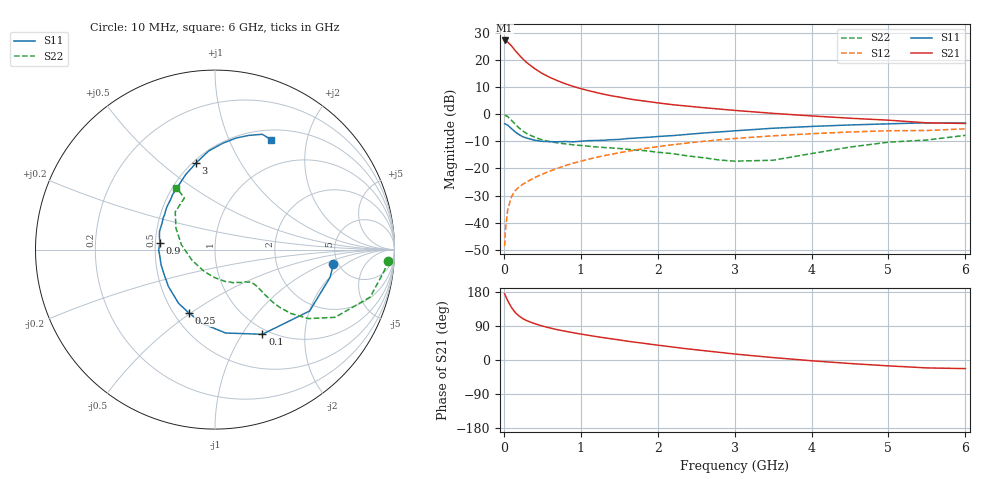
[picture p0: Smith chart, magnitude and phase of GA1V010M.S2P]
! Infineon Technologies  Discrete & RF Semiconductors
! BF775
! Si NPN RF Bipolar Junction Transistor in SOT23
! VCE = 1 V  IC = 10 mA
! Common Emitter S-Parameters:  May  1996
# GHz  S  MA  R  50
!  f  S11  S21  S12  S22
! GHz  MAG  ANG  MAG  ANG  MAG  ANG  MAG  ANG
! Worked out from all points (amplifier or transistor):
!   36 points, 10 MHz to 6 GHz, reference 50 ohm
!   highest |S21| = 27.2 dB at 10 MHz (marker M1)
!   |S21| within 3 dB of that: start of sweep to 127.4 MHz
!   unconditionally stable (mu >= 1): 472.2 MHz to end of sweep
!   at 250 MHz: K = 0.74, MSG = 23.0 dB, |S12| = -25.8 dB
!   at 1.4 GHz: K = 1.17, MAG = 8.3 dB, |S12| = -14.8 dB
!   at 6 GHz: K = 1.03, MAG = -0.1 dB, |S12| = -5.4 dB
!   S11 on the Smith chart (normalised r, x): 10 MHz: 4.56, -1.33; 100 MHz: 0.93, -1.23; 250 MHz: 0.59, -0.49; 900 MHz: 0.53, +0.05; 3 GHz: 0.52, +0.66; 6 GHz: 0.62, +1.44
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0.01  0.6648 -7.0  22.82 175.1  0.0037 87.6  0.9674 -3.6
0.02  0.6595 -13.6  22.5 170.1  0.0072 82.6  0.9509 -7.1
0.05  0.6283 -33.0  21.39 156.6  0.0174 75.3  0.9043 -17.0
0.1  0.5405 -60.8  18.06 138.4  0.0303 66.1  0.7684 -29.4
0.15  0.4685 -82.7  14.73 124.9  0.0395 59.9  0.6478 -36.4
0.2  0.4187 -99.4  12.27 115.7  0.0457 57.9  0.5541 -40.0
0.25  0.3814 -112.6  10.31 108.7  0.0515 57.3  0.485 -41.7
0.3  0.3616 -124.1  8.868 103.6  0.0568 57.6  0.4391 -42.3
0.4  0.3312 -141.5  6.917 95.9  0.0678 59.0  0.3764 -42.1
0.5  0.3153 -154.3  5.61 89.6  0.0786 59.8  0.3352 -41.5
0.6  0.3121 -164.4  4.753 84.5  0.0895 60.8  0.312 -41.2
0.7  0.3095 -172.5  4.12 79.8  0.1008 61.2  0.2961 -41.4
0.9  0.3091 172.8  3.253 72.0  0.1248 60.9  0.273 -42.2
1.1  0.3253 161.9  2.716 65.2  0.1479 60.1  0.2572 -44.8
1.3  0.3307 152.7  2.33 58.8  0.1716 58.6  0.2434 -47.7
1.6  0.3547 140.1  1.943 49.8  0.2064 55.5  0.2259 -54.2
2.2  0.4033 121.7  1.492 34.1  0.2742 48.4  0.187 -72.0
3  0.4932 102.5  1.174 15.8  0.3562 37.4  0.1363 -115.9
3.5  0.5513 93.6  1.035 6.4  0.3992 30.2  0.1417 -156.4
4.5  0.633 79.2  0.842 -9.3  0.4697 16.5  0.2477 151.4
5.5  0.6943 67.7  0.692 -20.9  0.5004 2.7  0.3344 120.7
6  0.6875 63.1  0.675 -22.7  0.5376 -1.3  0.4075 121.9
